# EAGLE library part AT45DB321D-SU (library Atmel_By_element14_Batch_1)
32-megabit DataFlash
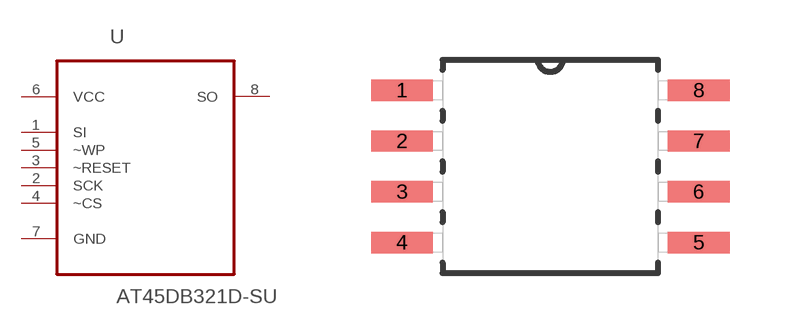
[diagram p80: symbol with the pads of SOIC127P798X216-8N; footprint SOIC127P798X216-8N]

Designator prefix U

## AT45DB321D-SU (MPN: AT45DB321D-SU; OC_FARNELL: 1455042; OC_NEWARK: 58M3840; PACKAGE: SOIC-8; SUPPLIER: ATMEL)  [SOIC127P798X216-8N]
1  SI  in
2  SCK  in
3  ~RESET  in
4  ~CS  in
5  ~WP  in
6  VCC  pwr
7  GND  pas
8  SO  out

## Footprint SOIC127P798X216-8N (pad centres in mm)
smd 1.549 x 0.533: 1 -3.708,1.905; 2 -3.708,0.635; 3 -3.708,-0.635; 4 -3.708,-1.905; 5 3.708,-1.905; 6 3.708,-0.635; 7 3.708,0.635; 8 3.708,1.905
